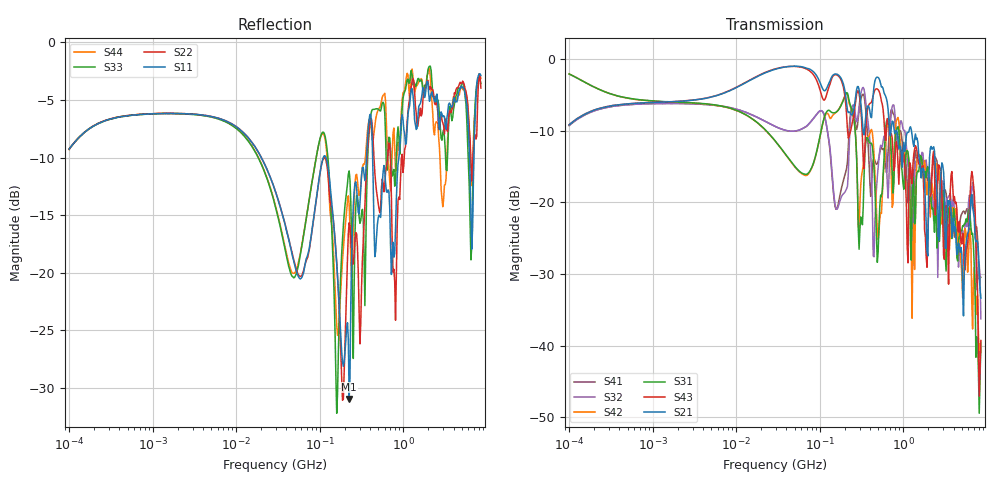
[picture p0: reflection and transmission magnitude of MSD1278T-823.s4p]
# MHz S MA R 50
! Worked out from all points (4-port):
!   498 points, 100 kHz to 8.5 GHz, reference 50 ohm
!   strongest paths, dB at 100 kHz, 1.698 MHz, 29.49 MHz, 500.7 MHz, 8.5 GHz:
!     S21: -9.2, -6.0, -1.4, -2.6, -33.4
!     S43: -9.2, -6.0, -1.4, -4.3, -39.3
!     S31: -2.1, -6.0, -11.5, -26.9, -39.5
!     S42: -2.1, -6.0, -11.5, -25.2, -40.9
!     S32: -9.3, -6.2, -9.4, -15.1, -36.3
!     S41: -9.3, -6.2, -9.4, -14.3, -30.5
!   lowest |S11| = -30.9 dB at 225.1 MHz (marker M1), VSWR 1.06, Z = 52.1 - j1.99 ohm
!   |S11| at or under -10 dB: 119 MHz to 363.6 MHz (244.6 MHz wide, 101 % of centre); 430 MHz to 887 MHz (457 MHz wide, 69.4 % of centre); 6.21 GHz to 7.012 GHz (802 MHz wide, 12.1 % of centre)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
0.1  0.3443 43.5  0.3463 44.5  0.7843 -18.1  0.3425 -136.2
     0.3463 44.5  0.3428 43.8  0.3432 -136.1  0.7849 -18.2
     0.7843 -18.1  0.3432 -136.1  0.3441 43.8  0.347 44.5
     0.3425 -136.2  0.7849 -18.2  0.347 44.5  0.3452 44.0
159.8183  0.1099 -119.4  0.7818 -39.6  0.428 43.9  0.08932 0.3
          0.7818 -39.6  0.1109 -110.7  0.08924 -5.6  0.4269 47.3
          0.428 43.9  0.08924 -5.6  0.02456 -32.1  0.773 -46.9
          0.08932 0.3  0.4269 47.3  0.773 -46.9  0.05898 -43.9
225.1135  0.02837 -42.3  0.4265 -54.0  0.5093 -34.5  0.3204 49.1
          0.4265 -54.0  0.1648 -16.0  0.2385 72.9  0.4878 -29.7
          0.5093 -34.5  0.2385 72.9  0.2768 -21.0  0.2881 -59.1
          0.3204 49.1  0.4878 -29.7  0.2881 -59.1  0.1986 -53.7
2062.915  0.5551 -168.0  0.2053 168.4  0.1412 110.2  0.09605 147.9
          0.2053 168.4  0.624 -167.8  0.1607 118.9  0.1051 122.0
          0.1412 110.2  0.1607 118.9  0.7886 -177.6  0.1086 -84.4
          0.09605 147.9  0.1051 122.0  0.1086 -84.4  0.7651 170.0
3821.877  0.5248 -8.1  0.0566 152.9  0.05582 -23.2  0.06908 -1.0
          0.0566 152.9  0.5107 -6.7  0.08006 -14.5  0.09176 -27.1
          0.05582 -23.2  0.08006 -14.5  0.4573 -15.1  0.1636 30.7
          0.06908 -1.0  0.09176 -27.1  0.1636 30.7  0.5176 1.7
6764.496  0.1568 75.6  0.09221 24.9  0.06062 22.0  0.1108 54.6
          0.09221 24.9  0.2914 70.6  0.1365 56.6  0.01306 -148.0
          0.06062 22.0  0.1365 56.6  0.2018 62.2  0.1522 16.2
          0.1108 54.6  0.01306 -148.0  0.1522 16.2  0.2743 97.7
8500  0.7182 -53.0  0.02148 -85.3  0.01056 -9.8  0.02994 -134.7
      0.02148 -85.3  0.6339 -46.1  0.01538 -147.2  0.008976 -142.8
      0.01056 -9.8  0.01538 -147.2  0.6633 -48.8  0.01085 -28.2
      0.02994 -134.7  0.008976 -142.8  0.01085 -28.2  0.6969 -49.0
